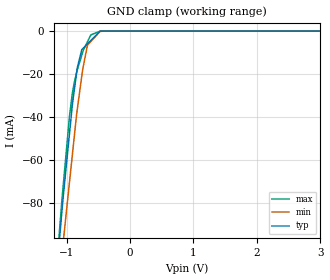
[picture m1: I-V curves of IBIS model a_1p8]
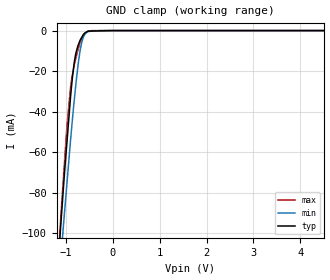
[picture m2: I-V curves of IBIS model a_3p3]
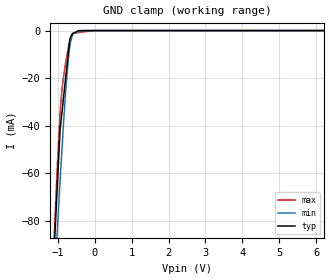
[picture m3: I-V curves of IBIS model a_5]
|Texas Instruments Incorporated
|Dual Buffer/Driver with Open-Drain Output
| Marketing part#   Digital Voltage Range   Package-type   #pins
| SN74LVC2G07DRYR   1.65V - 5.5V   SON   6
| SN74LVC2G07DSFR   1.65V - 5.5V   SON   6
| SN74LVC2G07DCKR   1.65V - 5.5V   SC70   6
| SN74LVC2G07DBVR   1.65V - 5.5V   SOT23   6
| SN74LVC2G07YZPR   1.65V - 5.5V   BGA   6
[IBIS Ver]   4.1
[File name]   sn74lvc2g07.ibs
[File Rev]   1.1
[Date]   1/6/2017
[Source]
| Texas Instruments Incorporated.
| Analog-eLab Design Center, HPA
| 12500 TI Blvd
| Dallas, TX -75243
| e-mail: elab_scm_ibis@list.ti.com
[Notes]   Revision History:
| Rev 1.1: 1/6/2017
| - Add package components DCK, DBV and YZP
| Rev 1.0: 6/26/2012
| - Initial version of the model
| - Model generated from simulations in TISPICE
| - Model matched to SPICE simulation
| - C_comp although listed in numerical order of value are
|   obtained from varying PVT conditions. For PVT conditions for
|   each specific value refer the buffer description under
|   respective [Model]. IBIS model user is responsible for using
|   appropriate C_comp to simulate for Signal Integrity.
| - Model names with a trailing _1p8 contains the model for
|   1.8V [1.71V and 1.89V]. Model names with a trailing _3p3
|   contains the model for 3.3V [3.0V and 3.6V]. Model names with
|   a trailing _5 contains the model for 5V [4.5V and 5.5V].
[Disclaimer]
| This model is designed as an aid for customers of Texas Instruments.
| TI and its licensors and suppliers make no warranties, either expressed
| or implied, with respect to this  model, including the warranties of
| merchantability or fitness for a particular purpose. The model is
| provided solely on an "as is" basis. The entire risk as to its quality
| and performance is with the customer.
[Copyright]
(C) Copyright 2012 Texas Instruments Incorporated.All rights reserved.
|   SN74LVC2G07DRY
[Component]   SN74LVC2G07DRY
[Manufacturer]   TI
[Package]   |6 SON   -  DRY package
|   typ   min   max
R_pkg   0.04713   0.04566   0.05129
L_pkg   0.47582nH   0.45735nH   0.52784nH
C_pkg   0.11172pF   0.11021pF   0.11567pF
[Pin]  signal_name   model_name   R_pin   L_pin   C_pin
1   1A   A   0.04566   0.46076nH  0.11062pF
2   GND   GND   0.04120   0.40932nH  0.10990pF
3   2A   A   0.05129   0.52784nH  0.11567pF
4   2Y   Y   0.04578   0.45735nH  0.11040pF
5   VCC   POWER   0.04120   0.40269nH  0.10933pF
6   1Y   Y   0.04578   0.45735nH  0.11021pF
|   SN74LVC2G07DSF
[Component]   SN74LVC2G07DSF
[Manufacturer]   TI
[Package]   |6 SON   -  DSF package
|   typ   min   max
R_pkg   0.04143   0.04038   0.04443
L_pkg   0.41914nH   0.39859nH   0.46140nH
C_pkg   0.10885pF   0.10755pF   0.11198pF
[Pin]  signal_name   model_name   R_pin   L_pin   C_pin
1   1A   A   0.04055   0.39859nH  0.10794pF
2   GND   GND   0.03830   0.39116nH  0.10996pF
3   2A   A   0.04443   0.46140nH  0.11198pF
4   2Y   Y   0.04038   0.40829nH  0.10793pF
5   VCC   POWER   0.03830   0.38405nH  0.10909pF
6   1Y   Y   0.04038   0.40828nH  0.10755pF
|   SN74LVC2G07DCK
[Component]   SN74LVC2G07DCK
[Manufacturer]   TI
[Package]   |6 SC70   -  DCK package
|   typ   min   max
R_pkg   0.0605   0.0578   0.0649
L_pkg   1.4789n   1.3445n   1.5572n
C_pkg   0.2188p   0.1428p   0.2401p
[Pin]  signal_name   model_name   R_pin   L_pin   C_pin
1   1A   A   0.05786  1.49630n  0.22530pF
2   GND   GND   0.05781  1.49553n  0.22752pF
3   2A   A   0.06185  1.55703n  0.24008pF
4   2Y   Y   0.05865  1.42253n  0.23839pF
5   VCC   POWER   0.06186  1.55724n  0.23889pF
6   1Y   Y   0.06494  1.34448n  0.14275pF
|   SN74LVC2G07DBV
[Component]   SN74LVC2G07DBV
[Manufacturer]   TI
[Package]   |6 SOT23   -  DBV package
|   typ   min   max
R_pkg   0.0792   0.0646   0.0861
L_pkg   1.8700n   1.5304n   2.0081n
C_pkg   0.2499p   0.2175p   0.2699p
[Pin]  signal_name   model_name   R_pin   L_pin   C_pin
1   1A   A   0.07690  1.85276n  0.25081pF
2   GND   GND   0.07719  1.85778n  0.24859pF
3   2A   A   0.08478  1.99126n  0.26602pF
4   2Y   Y   0.06461  1.53043n  0.24666pF
5   VCC   POWER   0.08591  2.00814n  0.26985pF
6   1Y   Y   0.08607  1.97934n  0.21754pF
|   SN74LVC2G07YZP
[Component]   SN74LVC2G07YZP
[Manufacturer]   TI
[Package]   |6 BGA   -  YZP package
|   typ   min   max
R_pkg   0.005   0.005   0.005
L_pkg   0.20nH   0.2nH   0.2nH
C_pkg   0.6pF   0.6pF   0.6pF
[Pin]  signal_name   model_name   R_pin   L_pin   C_pin
1   1A   A   0.005   0.2nH   0.6pF
2   GND   GND   0.005   0.2nH   0.6pF
3   2A   A   0.005   0.2nH   0.6pF
4   2Y   Y   0.005   0.2nH   0.6pF
5   VCC   POWER   0.005   0.2nH   0.6pF
6   1Y   Y   0.005   0.2nH   0.6pF
|   Model Selectors
[Model Selector] A
a_1p8   1.8V  digital input
a_3p3   3.3V  digital input
a_5   5.0V  digital input
[Model Selector] Y
y_1p8   1.8V  digital Open_drain
y_3p3   3.3V  digital Open_drain
y_5   5.0V  digital Open_drain
| Models and submodels in the file (6): a_1p8 (Input), a_3p3 (Input), a_5 (Input), y_1p8 (Open_drain), y_3p3 (Open_drain), y_5 (Open_drain)
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|   a_1p8 Model
[Model]   a_1p8
Model_type   Input
Vinl = 0.63
Vinh = 1.17
|   typ   min   max
|   (nom PVT)   (fast PVT)   (slow PVT)
|C_comp from frequency sweep method (F=10MHz)
|Average
|C_comp   3.427e-12   3.292e-12   6.436e-12
|C_comp from LC tank measurement(L=1nH)
|Average
|Resonant Frequency(Hz)   3.050e+09   3.070e+09   3.040e+09
C_comp   2.726e-12   2.690e-12   2.744e-12
[Model spec]
Vinl   0.63   0.599   0.662
Vinh   1.17   1.112   1.229
| Where nom  PVT is Nominal Process, 1.8V, 27C
|   Fast PVT is Strong Process,  1.89V, -40C
|   Slow PVT is Weak Process,   1.71V, 125C
[Voltage Range]   1.8   1.71   1.89
|Ambient Temperature   25   85   -40
|Junction Temperature
[Temperature Range]   27   125   -40
[Power Clamp Reference]   1.8   1.71   1.89
[GND Clamp Reference]   0   0   0
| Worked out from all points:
|   GND clamp passes 1 mA (typ) near -0.50 V on its own axis
[GND Clamp]
|   Voltage   I(typ)   I(min)   I(max)
-1.8V     -348.5mA   -332.5mA   -371.8mA
-1.206V   -129.1mA   -141.6mA   -129mA
-1.075V   -85mA      -104.9mA   -79.74mA
-1.055V   -78.02mA   -99.05mA   -72.96mA
-952.6mV  -47.57mA   -70.22mA   -39.53mA
-907.2mV  -34.12mA   -57.42mA   -28.82mA
-831.6mV  -17.29mA   -36.74mA   -18.23mA
-759.6mV  -8.64mA    -20.93mA   -11.23mA
-670.3mV  -5.985mA   -6.607mA   -5.006mA
-616.1mV  -4.373mA   -4.859mA   -1.764mA
-424.1mV  -35.63uA   -56.93uA   -7.59uA
3.6V      0A         0A         0A
[POWER Clamp]
|   Voltage   I(typ)   I(min)   I(max)
-1.8V     0A         0A         0A
0V        0A         0A         0A
3.6V      0A         0A         0A
|   a_3p3 Model
[Model]   a_3p3
Model_type   Input
Vinl = 0.8
Vinh = 2
|   typ   min   max
|   (nom PVT)   (fast PVT)   (slow PVT)
|C_comp from frequency sweep method (F=10MHz)
|Average
|C_comp   3.480e-12   3.309e-12   3.701e-12
|C_comp from LC tank measurement(L=1nH)
|Average
|Resonant Frequency(Hz)   3.120e+09   3.120e+09   3.110e+09
C_comp   2.605e-12   2.605e-12   2.622e-12
| Where nom  PVT is Nominal Process, 3.3V, 27C
|   Fast PVT is Strong Process,  3.6V, -40C
|   Slow PVT is Weak Process,   3V, 125C
[Voltage Range]   3.3   3   3.6
|Ambient Temperature   25   85   -40
|Junction Temperature
[Temperature Range]   27   125   -40
[Power Clamp Reference]   3.3   3   3.6
[GND Clamp Reference]   0   0   0
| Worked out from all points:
|   GND clamp passes 1 mA (typ) near -0.58 V on its own axis
[GND Clamp]
|   Voltage   I(typ)   I(min)   I(max)
-3.3V     -951.6mA   -864.1mA   -1.023A
-1.218V   -132.8mA   -145.3mA   -133.8mA
-1.109V   -95.69mA   -112.8mA   -91.88mA
-1.059V   -79.51mA   -97.93mA   -74.7mA
-979.2mV  -55.41mA   -75.8mA    -47.3mA
-896.4mV  -31.37mA   -52.85mA   -26.85mA
-818.4mV  -15.14mA   -33.59mA   -16.84mA
-738mV    -7.17mA    -16.45mA   -9.122mA
-663mV    -3.386mA   -5.871mA   -4.219mA
-591mV    -1.096mA   -1.64mA    -1.334mA
-522mV    -261.2uA   -440.6uA   -180.9uA
6.6V      0A         0A         0A
[POWER Clamp]
|   Voltage   I(typ)   I(min)   I(max)
-3.3V     0A         0A         0A
0V        0A         0A         0A
6.6V      0A         0A         0A
|   a_5 Model
[Model]   a_5
Model_type   Input
Vinl = 1.5
Vinh = 3.5
|   typ   min   max
|   (nom PVT)   (fast PVT)   (slow PVT)
|C_comp from frequency sweep method (F=10MHz)
|Average
|C_comp   4.239e-12   3.909e-12   4.636e-12
|C_comp from LC tank measurement(L=1nH)
|Average
|Resonant Frequency(Hz)   3.160e+09   3.170e+09   3.160e+09
C_comp   2.539e-12   2.523e-12   2.539e-12
[Model spec]
Vinl   1.5   1.35   1.65
Vinh   3.5   3.15   3.85
| Where nom  PVT is Nominal Process, 5V, 27C
|   Fast PVT is Strong Process,  5.5V, -40C
|   Slow PVT is Weak Process,   4.5V, 125C
[Voltage Range]   5   4.5   5.5
|Ambient Temperature   25   85   -40
|Junction Temperature
[Temperature Range]   27   125   -40
[Power Clamp Reference]   5   4.5   5.5
[GND Clamp Reference]   0   0   0
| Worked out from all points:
|   GND clamp passes 1 mA (typ) near -0.56 V on its own axis
[GND Clamp]
|   Voltage   I(typ)   I(min)   I(max)
-5V       -1.655A    -1.496A    -1.772A
-1.089V   -90.09mA   -106.7mA   -84.64mA
-1.067V   -83.01mA   -100.1mA   -76.85mA
-1.062V   -81.6mA    -98.8mA    -75.3mA
-1.001V   -62.41mA   -81.63mA   -54.18mA
-935mV    -41.65mA   -63.18mA   -34.94mA
-874.5mV  -32.94mA   -47.55mA   -23.48mA
-760.5mV  -16.54mA   -20.76mA   -11.36mA
-670.5mV  -3.588mA   -6.626mA   -4.372mA
-576mV    -1.163mA   -1.241mA   -1.09mA
-435mV    -28.12uA   -492.2uA   -823.1uA
10V       0A         0A         0A
[POWER Clamp]
|   Voltage   I(typ)   I(min)   I(max)
-5V       0A         0A         0A
0V        0A         0A         0A
10V       0A         0A         0A
